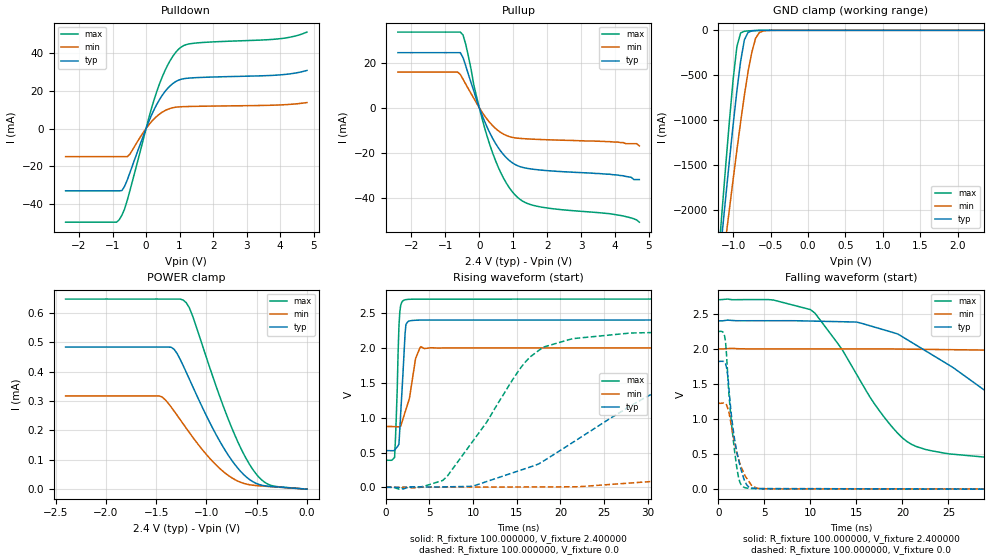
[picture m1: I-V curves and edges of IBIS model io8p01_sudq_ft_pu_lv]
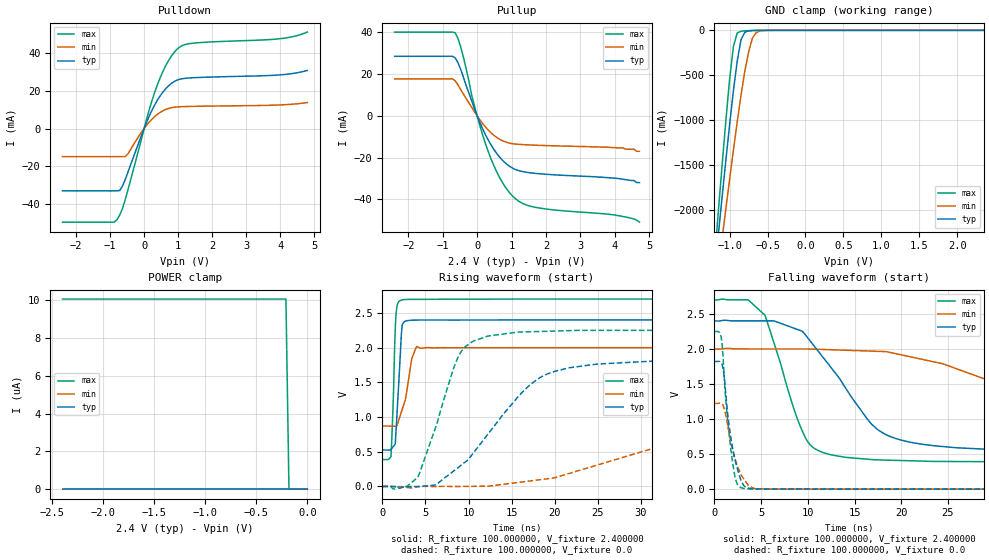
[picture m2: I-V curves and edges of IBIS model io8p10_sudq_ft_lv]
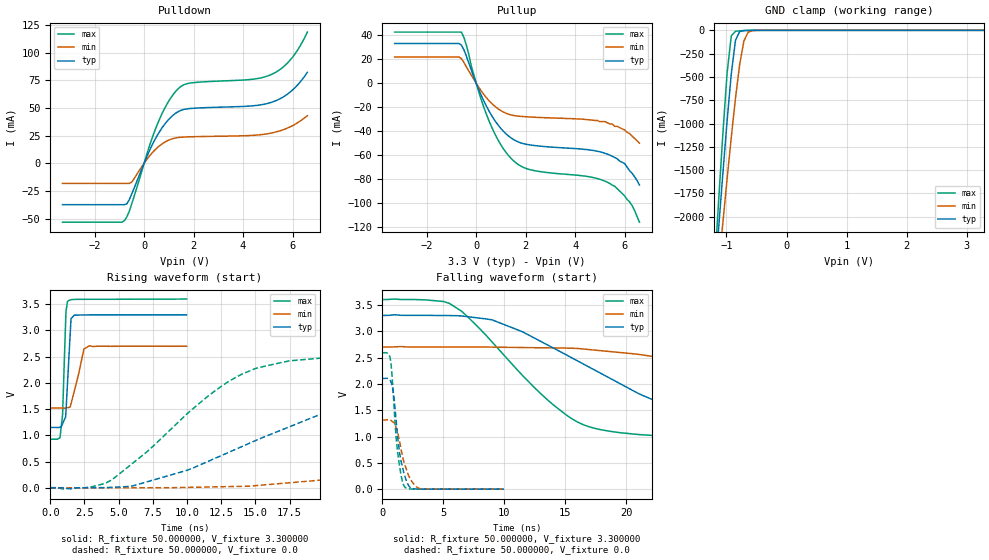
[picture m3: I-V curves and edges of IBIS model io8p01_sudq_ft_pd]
| IBIS file stm32f303x6x8_334_wlcsp49.ibs
[IBIS ver] 4.2
[File name] stm32f303x6x8_334_wlcsp49.ibs
[File Rev] 1
[Date]  29-09-2025
[Source] Data Created at STMicroelectronics
[Notes]  File originated from ELDO simulations.
[Disclaimer]  This information is for modeling purpose only and is
   not guaranted. The information is subject to change without
   notice.
[Copyright] Copyright 2025 STMicroelectronics Inc.
|   Component stm32f303x6x8_334_wlcsp49
[Component] stm32f303x6x8_334_wlcsp49
[Manufacturer] STMicroelectronics
[Package]
| variable   typ   min   max
R_pkg   0.0   0.0   0.0
L_pkg   0.0H   0.0H   0.0H
C_pkg   0.0F   0.0F   0.0F
[Pin]  signal_name   model_name   R_pin   L_pin   C_pin
A1 PA14 io8p_wsudqh_i2c_ft
A2 PA15 io8p_wsudqh_i2c_ft
A3 PB3 io8p_sudq_ft
A4 PB6 io8p_wsudqh_i2c_ft
A5 BOOT0 vpp_test_hv
A6 PB9 io8p_wsudqh_i2c_ft
A7 VDD POWER
B1 VSS GND
B2 VDD POWER
B3 PB4 io8p_sudq_ft
B4 PB5 io8p_sudq_ft
B5 PB7 io8p_wsudqh_i2c_ft
B6 PB8 io8p_wsudqh_i2c_ft
B7 VSS GND
C1 PA11 io8p_sudq_ft
C2 PA13 io8p_sudq_ft
C3 PA12 io8p_sudq_ft
C4 PA10 io8p_sudq_ft
C5 PC3 io8p_sudq_tc
C6 PF1 io8p_sudq_ft
C7 PF0 io8p_sudq_ft
D1 PA8 io8p_sudq_ft
D2 PA9 io8p_sudq_ft
D3 PB15 io8p_sudq_tc
D4 PC7 io8p_sudq_ft
D5 PA2 io8p_sudq_tc
D6 PA0 io8p_sudq_tc
D7 NRST ioreset_tc_v33
E1 PB14 io8p_sudq_tc
E2 PB13 io8p_sudq_tc
E3 PC5 io8p_sudq_tc
E4 PA6 io8p_sudq_tc
E5 PA3 io8p_sudq_tc
E6 VDDA POWER
E7 VSSA GND
F1 PB12 io8p_sudq_tc
F2 PB2 io8p_sudq_tc
F3 PB0 io8p_sudq_tc
F4 PA7 io8p_sudq_tc
F5 PA4 io8p_sudq_tc
F6 VSS GND
F7 VREFP POWER
G1 PB11 io8p_sudq_tc
G2 PB10 io8p_sudq_tc
G3 PB1 io8p_sudq_tc
G4 PC4 io8p_sudq_tc
G5 PA5 io8p_sudq_tc
G6 VDD POWER
G7 PA1 io8p_sudq_tc
[Model Selector] io8p_sudq_ft
io8p01_sudq_ft_pd_lv  "SPEED01 2P0V, PD=40kOhm"
io8p01_sudq_ft_pu_lv  "SPEED01 2P0V, PU=40kOhm"
io8p01_sudq_ft_lv  "SPEED01 2P0V"
io8p10_sudq_ft_pd_lv  "SPEED10 2P0V, PD=40kOhm"
io8p10_sudq_ft_pu_lv  "SPEED10 2P0V, PU=40kOhm"
io8p10_sudq_ft_lv  "SPEED10 2P0V"
io8p11_sudq_ft_pd_lv  "SPEED11 2P0V, PD=40kOhm"
io8p11_sudq_ft_pu_lv  "SPEED11 2P0V, PU=40kOhm"
io8p11_sudq_ft_lv  "SPEED11 2P0V"
io8p01_sudq_ft_pd  "SPEED01, PD=40kOhm"
io8p01_sudq_ft_pu  "SPEED01, PU=40kOhm"
io8p01_sudq_ft  "SPEED01"
io8p10_sudq_ft_pd  "SPEED10, PD=40kOhm"
io8p10_sudq_ft_pu  "SPEED10, PU=40kOhm"
io8p10_sudq_ft  "SPEED10"
io8p11_sudq_ft_pd  "SPEED11, PD=40kOhm"
io8p11_sudq_ft_pu  "SPEED11, PU=40kOhm"
io8p11_sudq_ft  "SPEED11"
[Model Selector] io8p_sudq_tc
io8p01_sudq_tc_pd_lv  "SPEED01 2P0V, PD=40kOhm"
io8p01_sudq_tc_pu_lv  "SPEED01 2P0V, PU=40kOhm"
io8p01_sudq_tc_lv  "SPEED01 2P0V"
io8p10_sudq_tc_pd_lv  "SPEED10 2P0V, PD=40kOhm"
io8p10_sudq_tc_pu_lv  "SPEED10 2P0V, PU=40kOhm"
io8p10_sudq_tc_lv  "SPEED10 2P0V"
io8p11_sudq_tc_pd_lv  "SPEED11 2P0V, PD=40kOhm"
io8p11_sudq_tc_pu_lv  "SPEED11 2P0V, PU=40kOhm"
io8p11_sudq_tc_lv  "SPEED11 2P0V"
io8p01_sudq_tc_pd  "SPEED01, PD=40kOhm"
io8p01_sudq_tc_pu  "SPEED01, PU=40kOhm"
io8p01_sudq_tc  "SPEED01"
io8p10_sudq_tc_pd  "SPEED10, PD=40kOhm"
io8p10_sudq_tc_pu  "SPEED10, PU=40kOhm"
io8p10_sudq_tc  "SPEED10"
io8p11_sudq_tc_pd  "SPEED11, PD=40kOhm"
io8p11_sudq_tc_pu  "SPEED11, PU=40kOhm"
io8p11_sudq_tc  "SPEED11"
[Model Selector] io8p_wsudqh_i2c_ft
io8p_wsudqh_i2c_ft_lv_pd  "General purpose IO with I2C capability on. 5V tolerant. 1.8V range with pull down"
io8p_wsudqh_i2c_ft_lv_pu  "General purpose IO with I2C capability on. 5V tolerant. 1.8V range with pull up"
io8p_wsudqh_i2c_ft_lv  "General purpose IO with I2C capability on. 5V tolerant. 1.8V range"
io8p_wsudqh_i2c_ft_pd  "General purpose IO with I2C capability on. 5V tolerant. 3.3V range with pull down"
io8p_wsudqh_i2c_ft_pu  "General purpose IO with I2C capability on. 5V tolerant. 3.3V range with pull up"
io8p_wsudqh_i2c_ft_i2c  "General purpose IO with I2C capability on. 5V tolerant. 3.3V range"
[Model Selector] ioreset_tc_v33
ioreset_tc_v33_pu_lv  "IORESET 2V + PU=40kOhm"
ioreset_tc_v33_nopu_lv  "IORESET 2V"
ioreset_tc_v33_pu  "IORESET + PU=40kOhm"
ioreset_tc_v33_nopu  "IORESET"
[Model Selector] vpp_test_hv
vpp_test_hv_3p3  "Input Buffer"
vpp_test_hv_2p4  "Input Buffer 2P0V"
| Models and submodels in the file (48): io8p01_sudq_ft_pd_lv (I/O), io8p01_sudq_ft_pu_lv (I/O), io8p01_sudq_ft_lv (I/O), io8p10_sudq_ft_pd_lv (I/O), io8p10_sudq_ft_pu_lv (I/O), io8p10_sudq_ft_lv (I/O), io8p11_sudq_ft_pd_lv (I/O), io8p11_sudq_ft_pu_lv (I/O), io8p11_sudq_ft_lv (I/O), io8p01_sudq_ft_pd (I/O), io8p01_sudq_ft_pu (I/O), io8p01_sudq_ft (I/O), io8p10_sudq_ft_pd (I/O), io8p10_sudq_ft_pu (I/O), io8p10_sudq_ft (I/O), io8p11_sudq_ft_pd (I/O), io8p11_sudq_ft_pu (I/O), io8p11_sudq_ft (I/O), io8p01_sudq_tc_pd_lv (I/O), io8p01_sudq_tc_pu_lv (I/O), io8p01_sudq_tc_lv (I/O), io8p10_sudq_tc_pd_lv (I/O), io8p10_sudq_tc_pu_lv (I/O), io8p10_sudq_tc_lv (I/O), io8p11_sudq_tc_pd_lv (I/O), io8p11_sudq_tc_pu_lv (I/O), io8p11_sudq_tc_lv (I/O), io8p01_sudq_tc_pd (I/O), io8p01_sudq_tc_pu (I/O), io8p01_sudq_tc (I/O), io8p10_sudq_tc_pd (I/O), io8p10_sudq_tc_pu (I/O), io8p10_sudq_tc (I/O), io8p11_sudq_tc_pd (I/O), io8p11_sudq_tc_pu (I/O), io8p11_sudq_tc (I/O), io8p_wsudqh_i2c_ft_lv_pd (I/O), io8p_wsudqh_i2c_ft_lv_pu (I/O), io8p_wsudqh_i2c_ft_lv (I/O), io8p_wsudqh_i2c_ft_pd (I/O), io8p_wsudqh_i2c_ft_pu (I/O), io8p_wsudqh_i2c_ft_i2c (I/O), ioreset_tc_v33_pu_lv (I/O_open_drain), ioreset_tc_v33_nopu_lv (I/O_open_drain), ioreset_tc_v33_pu (I/O_open_drain), ioreset_tc_v33_nopu (I/O_open_drain), vpp_test_hv_2p4 (Input), vpp_test_hv_3p3 (Input)
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|   Model io8p01_sudq_ft_pu_lv
[Model]  io8p01_sudq_ft_pu_lv
Model_type I/O
Polarity   Non-Inverting
Enable   Active-Low
Vinl =   0.720000V
Vinh =   1.680000V
Vmeas =  1.200000V
Cref =   50.000000pF
Rref =   100.000000M
Vref =   0.0V
C_comp   1.970100pF   1.887900pF   2.069400pF
[Temperature Range]   25.000000   0.125000k   -40.000000
[Pullup Reference]   2.400000V   2.000000V   2.700000V
[Pulldown Reference]   0.0V   0.0V   0.0V
[POWER Clamp Reference]   2.400000V   2.000000V   2.700000V
[GND Clamp Reference]   0.0V   0.0V   0.0V
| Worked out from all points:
|   slope of the pulldown table from 0 to 0.36 V, typ, clamps not added: 25.5 ohm
|   slope of the pullup table from 0 to 0.36 V, typ, clamps not added: 28.4 ohm
|   GND clamp passes 1 mA (typ) near -0.64 V on its own axis
|   rising waveform, R_fixture 100.000000, V_fixture 2.400000: 20-80 % time 497ps typ, 1.06ns min, 335ps max; typ from 0.527 V to 2.4 V
|   rising waveform, R_fixture 100.000000, V_fixture 0.0: 20-80 % time 14.6ns typ, 42.8ns min, 7.27ns max; typ from 0.001 V to 1.82 V
|   falling waveform, R_fixture 100.000000, V_fixture 2.400000: 20-80 % time 12.9ns typ, 32.5ns min, 7.06ns max; typ from 2.4 V to 0.527 V
|   falling waveform, R_fixture 100.000000, V_fixture 0.0: 20-80 % time 1.16ns typ, 1.4ns min, 913ps max; typ from 1.82 V to 0.001 V
[Pulldown]
|Voltage   I(typ)   I(min)   I(max)
-2.4V     -33.16mA   -14.98mA   -49.86mA
-880mV    -33.16mA   -14.98mA   -49.86mA
-800mV    -33.16mA   -14.98mA   -48.55mA
-640mV    -30.75mA   -14.98mA   -42.77mA
-480mV    -23.43mA   -13.57mA   -32.92mA
80mV      3.651mA    1.905mA    5.506mA
400mV     15.37mA    7.665mA    23.73mA
720mV     22.75mA    10.69mA    36.23mA
1.04V     26.18mA    11.57mA    43.27mA
1.52V     27.09mA    11.81mA    45.55mA
4V        28.55mA    12.55mA    47.81mA
4.8V      30.9mA     13.81mA    51.31mA
[Pullup]
|Voltage   I(typ)   I(min)   I(max)
-2.4V     24.57mA    15.91mA    33.73mA
-640mV    24.57mA    15.91mA    33.73mA
-480mV    22.32mA    12.71mA    32.43mA
-400mV    18.71mA    10.52mA    28.28mA
-160mV    7.421mA    4.162mA    10.02mA
0V        81fA       15.2pA     0A
320mV     -11.51mA   -6.781mA   -16.98mA
720mV     -21mA      -11.8mA    -31.53mA
1.2V      -26.24mA   -13.65mA   -40.83mA
1.76V     -27.69mA   -14.12mA   -44.07mA
3.84V     -29.6mA    -15.1mA    -47.2mA
4.72V     -32mA      -17mA      -51mA
[GND_clamp]
|Voltage   I(typ)   I(min)   I(max)
-2.4V     -9.788A    -9.782A    -9.734A
-1.2V     -2.718A    -3.02A     -2.568A
-1.15V    -2.29A     -2.675A    -2.036A
-1.1V     -1.868A    -2.333A    -1.515A
-1.05V    -1.454A    -1.995A    -1.012A
-950mV    -674.5mA   -1.337A    -180.5mA
-900mV    -345.2mA   -1.023A    -29.72mA
-850mV    -106.4mA   -726mA     -10.13mA
-750mV    -6.396mA   -244mA     -4.026mA
-700mV    -2.558mA   -88.61mA   -2.329mA
-600mV    -416uA     -7.739mA   -368uA
2.35V     0A         0A         0A
[POWER_clamp]
|Voltage   I(typ)   I(min)   I(max)
-2.4V     483.8uA    317.4uA    647uA
-1.47V    483.8uA    317.4uA    647uA
-1.32V    475.6uA    265.2uA    647uA
-1.23V    419.7uA    221.6uA    643.3uA
-1.17V    374.8uA    192.7uA    617.6uA
-1.14V    352.1uA    178.7uA    591.9uA
-840mV    147uA      62.15uA    289.6uA
-690mV    72.24uA    27.76uA    162.7uA
-540mV    25.74uA    13.55uA    67.63uA
-450mV    13.38uA    10.75uA    31.36uA
-360mV    9.231uA    8.535uA    12.97uA
0V        0A         0A         0A
[Ramp]
| variable   typ   min   max
dV/dt_r  1.09269/14.55881n   0.73353/42.71845n   1.34908/7.26325n
dV/dt_f  1.12400/12.83842n   0.67649/32.44923n   1.38689/7.04961n
R_load = 100.000000
[Rising Waveform]
R_fixture= 100.000000
V_fixture= 2.400000
V_fixture_min= 2.000000
V_fixture_max= 2.700000
|time   V(typ)   V(min)   V(max)
0s        526.5mV    872.5mV    388.6mV
1.001ns   534.8mV    870.7mV    429.3mV
1.301ns   581.8mV    869.1mV    1.401V
1.502ns   620.7mV    868.5mV    2.316V
1.602ns   841mV      868.2mV    2.522V
2.102ns   1.968V     1.038V     2.685V
2.302ns   2.337V     1.118V     2.692V
3.403ns   2.396V     1.846V     2.698V
4.004ns   2.398V     2.018V     2.698V
49.85ns   2.4V       2V         2.7V
[Rising Waveform]
R_fixture= 100.000000
V_fixture= 0.0
V_fixture_min= 0.0
V_fixture_max= 0.0
|time   V(typ)   V(min)   V(max)
0s        1.057mV    1.357mV    941.6uV
6.507ns   6.739mV    4.851mV    98.8mV
15.52ns   249.4mV    5.766mV    1.725V
18.02ns   374.6mV    6.657mV    2.009V
28.03ns   1.166V     62.6mV     2.213V
34.53ns   1.553V     120.9mV    2.23V
43.04ns   1.725V     229mV      2.248V
79.08ns   1.822V     883.8mV    2.25V
103.1ns   1.822V     1.116V     2.249V
249.2ns   1.822V     1.224V     2.25V
[Falling Waveform]
R_fixture= 100.000000
V_fixture= 2.400000
V_fixture_min= 2.000000
V_fixture_max= 2.700000
|time   V(typ)   V(min)   V(max)
0s        2.4V       2V         2.7V
10.01ns   2.397V     2V         2.56V
15.02ns   2.383V     2V         1.64V
20.02ns   2.171V     1.997V     729.2mV
29.53ns   1.353V     1.982V     451.1mV
38.04ns   762.8mV    1.926V     413.2mV
57.06ns   576.4mV    1.555V     391.8mV
84.58ns   537.8mV    1.049V     388.5mV
102.6ns   530.3mV    958.5mV    388.5mV
249.2ns   526.5mV    872.5mV    388.6mV
[Falling Waveform]
R_fixture= 100.000000
V_fixture= 0.0
V_fixture_min= 0.0
V_fixture_max= 0.0
|time   V(typ)   V(min)   V(max)
0s        1.822V     1.224V     2.25V
700.7ps   1.803V     1.224V     2.18V
800.8ps   1.785V     1.217V     2.098V
1.001ns   1.655V     1.167V     1.705V
1.401ns   1.091V     924.7mV    994.1mV
1.802ns   692.7mV    650.1mV    517.8mV
2.302ns   370.4mV    389.6mV    121.1mV
2.903ns   110.3mV    193.7mV    21.86mV
4.605ns   7.762mV    8.133mV    8.175mV
49.85ns   1.057mV    1.357mV    941.6uV
|   Model io8p10_sudq_ft_lv
[Model]  io8p10_sudq_ft_lv
Model_type I/O
Polarity   Non-Inverting
Enable   Active-Low
Vinl =   0.720000V
Vinh =   1.680000V
Vmeas =  1.200000V
Cref =   50.000000pF
Rref =   100.000000M
Vref =   0.0V
C_comp   1.970100pF   1.887900pF   2.069400pF
[Temperature Range]   25.000000   0.125000k   -40.000000
[Pullup Reference]   2.400000V   2.000000V   2.700000V
[Pulldown Reference]   0.0V   0.0V   0.0V
[POWER Clamp Reference]   2.400000V   2.000000V   2.700000V
[GND Clamp Reference]   0.0V   0.0V   0.0V
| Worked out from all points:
|   slope of the pulldown table from 0 to 0.36 V, typ, clamps not added: 25.5 ohm
|   slope of the pullup table from 0 to 0.36 V, typ, clamps not added: 28.4 ohm
|   GND clamp passes 1 mA (typ) near -0.64 V on its own axis
|   rising waveform, R_fixture 100.000000, V_fixture 2.400000: 20-80 % time 501ps typ, 1.06ns min, 336ps max; typ from 0.525 V to 2.4 V
|   rising waveform, R_fixture 100.000000, V_fixture 0.0: 20-80 % time 7.32ns typ, 21.7ns min, 3.52ns max; typ from 0 V to 1.82 V
|   falling waveform, R_fixture 100.000000, V_fixture 2.400000: 20-80 % time 6.27ns typ, 18.5ns min, 3.33ns max; typ from 2.4 V to 0.525 V
|   falling waveform, R_fixture 100.000000, V_fixture 0.0: 20-80 % time 1.16ns typ, 1.4ns min, 914ps max; typ from 1.82 V to 0 V
[Pulldown]
|Voltage   I(typ)   I(min)   I(max)
-2.4V     -33.16mA   -14.98mA   -49.86mA
-880mV    -33.16mA   -14.98mA   -49.86mA
-800mV    -33.16mA   -14.98mA   -48.55mA
-640mV    -30.75mA   -14.98mA   -42.76mA
-480mV    -23.43mA   -13.57mA   -32.92mA
80mV      3.651mA    1.905mA    5.506mA
400mV     15.37mA    7.665mA    23.73mA
720mV     22.75mA    10.69mA    36.23mA
1.04V     26.18mA    11.57mA    43.27mA
1.52V     27.09mA    11.81mA    45.55mA
4V        28.55mA    12.55mA    47.81mA
4.8V      30.9mA     13.81mA    51.31mA
[Pullup]
|Voltage   I(typ)   I(min)   I(max)
-2.4V     28.57mA    17.75mA    40.17mA
-720mV    28.57mA    17.75mA    40.17mA
-640mV    27.85mA    16.83mA    39.88mA
-480mV    22.38mA    12.65mA    33.22mA
-80mV     3.427mA    2.066mA    4.957mA
160mV     -6.219mA   -3.715mA   -9.137mA
320mV     -11.51mA   -6.781mA   -16.98mA
720mV     -21mA      -11.8mA    -31.54mA
1.12V     -25.77mA   -13.54mA   -39.82mA
1.76V     -27.69mA   -14.12mA   -44.07mA
4V        -29.9mA    -15.2mA    -47.5mA
4.72V     -32mA      -17mA      -51mA
[GND_clamp]
|Voltage   I(typ)   I(min)   I(max)
-2.4V     -9.788A    -9.782A    -9.734A
-1.2V     -2.718A    -3.02A     -2.568A
-1.15V    -2.29A     -2.675A    -2.036A
-1.1V     -1.868A    -2.333A    -1.515A
-1.05V    -1.454A    -1.995A    -1.012A
-950mV    -674.5mA   -1.337A    -180.5mA
-900mV    -345.2mA   -1.023A    -29.72mA
-850mV    -106.4mA   -726mA     -10.13mA
-750mV    -6.396mA   -244mA     -4.026mA
-700mV    -2.558mA   -88.61mA   -2.329mA
-600mV    -416uA     -7.739mA   -368uA
2.35V     0A         0A         0A
[POWER_clamp]
|Voltage   I(typ)   I(min)   I(max)
-2.4V     0A         0A         10.06uA
-210mV    0A         0A         10.06uA
-180mV    0A         0A         0A
0V        0A         0A         0A
[Ramp]
| variable   typ   min   max
dV/dt_r  1.09308/7.31082n   0.73308/21.71145n   1.34964/3.51759n
dV/dt_f  1.12481/6.26349n   0.67631/18.49686n   1.38754/3.32485n
R_load = 100.000000
[Rising Waveform]
R_fixture= 100.000000
V_fixture= 2.400000
V_fixture_min= 2.000000
V_fixture_max= 2.700000
|time   V(typ)   V(min)   V(max)
0s        525.2mV    870.3mV    387.4mV
1.001ns   533.2mV    868.7mV    426.9mV
1.301ns   579.1mV    867.1mV    1.388V
1.502ns   617.1mV    866.5mV    2.304V
1.702ns   1.054V     877mV      2.604V
2.202ns   2.189V     1.072V     2.684V
2.603ns   2.379V     1.227V     2.693V
3.403ns   2.395V     1.838V     2.696V
4.004ns   2.397V     2.017V     2.696V
49.85ns   2.4V       2V         2.7V
[Rising Waveform]
R_fixture= 100.000000
V_fixture= 0.0
V_fixture_min= 0.0
V_fixture_max= 0.0
|time   V(typ)   V(min)   V(max)
0s        1.81nV     16.19nV    1.388nV
2.803ns   -3.281mV   -14.07mV   -1.578mV
4.204ns   -1.834mV   -2.504mV   153.3mV
8.809ns   274.6mV    -1.375mV   1.87V
12.21ns   748.9mV    4.656mV    2.166V
18.02ns   1.547V     92.84mV    2.232V
24.82ns   1.763V     304.5mV    2.249V
40.24ns   1.817V     861.6mV    2.249V
51.85ns   1.822V     1.107V     2.249V
99.7ns    1.822V     1.223V     2.249V
[Falling Waveform]
R_fixture= 100.000000
V_fixture= 2.400000
V_fixture_min= 2.000000
V_fixture_max= 2.700000
|time   V(typ)   V(min)   V(max)
0s        2.4V       2V         2.7V
3.604ns   2.401V     2V         2.703V
5.405ns   2.402V     2V         2.482V
9.81ns    2.189V     2V         715.2mV
14.01ns   1.448V     1.982V     453.6mV
18.22ns   786.7mV    1.963V     414.6mV
25.83ns   591.3mV    1.722V     393.9mV
36.04ns   545.2mV    1.277V     387.5mV
53.05ns   528.1mV    942.3mV    387.4mV
99.7ns    525.2mV    870.3mV    387.4mV
[Falling Waveform]
R_fixture= 100.000000
V_fixture= 0.0
V_fixture_min= 0.0
V_fixture_max= 0.0
|time   V(typ)   V(min)   V(max)
0s        1.822V     1.223V     2.249V
700.7ps   1.802V     1.222V     2.18V
800.8ps   1.785V     1.215V     2.098V
1.001ns   1.656V     1.165V     1.707V
1.401ns   1.093V     924.2mV    997.1mV
1.902ns   616.8mV    592mV      421.8mV
2.302ns   368.5mV    388.7mV    122.4mV
2.903ns   107.4mV    191.2mV    17.72mV
4.705ns   2.748mV    4.47mV     1.93mV
49.85ns   1.81nV     16.19nV    1.388nV
|   Model io8p01_sudq_ft_pd
[Model]  io8p01_sudq_ft_pd
Model_type I/O
Polarity   Non-Inverting
Enable   Active-Low
Vinl =   0.990000V
Vinh =   2.310000V
Vmeas =  1.650000V
Cref =   50.000000pF
Rref =   100.000000M
Vref =   0.0V
C_comp   1.970900pF   1.892300pF   2.063200pF
[Temperature Range]   25.000000   0.125000k   -40.000000
[Pullup Reference]   3.300000V   2.700000V   3.600000V
[Pulldown Reference]   0.0V   0.0V   0.0V
[POWER Clamp Reference]   3.300000V   2.700000V   3.600000V
[GND Clamp Reference]   0.0V   0.0V   0.0V
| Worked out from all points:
|   slope of the pulldown table from 0 to 0.495 V, typ, clamps not added: 20.9 ohm
|   slope of the pullup table from 0 to 0.495 V, typ, clamps not added: 22.2 ohm
|   GND clamp passes 1 mA (typ) near -0.64 V on its own axis
|   rising waveform, R_fixture 50.000000, V_fixture 3.300000: 20-80 % time 269ps typ, 640ps min, 200ps max; typ from 1.15 V to 3.3 V
|   rising waveform, R_fixture 50.000000, V_fixture 0.0: 20-80 % time 12.6ns typ, 30.4ns min, 7.07ns max; typ from 0 V to 2.1 V
|   falling waveform, R_fixture 50.000000, V_fixture 3.300000: 20-80 % time 11ns typ, 22.7ns min, 6.9ns max; typ from 3.3 V to 1.15 V
|   falling waveform, R_fixture 50.000000, V_fixture 0.0: 20-80 % time 664ps typ, 860ps min, 541ps max; typ from 2.1 V to 0 V
[Pulldown]
|Voltage   I(typ)   I(min)   I(max)
-3.3V     -37.45mA   -18.2mA    -53.24mA
-800mV    -37.45mA   -18.2mA    -51.9mA
-700mV    -36.7mA    -18.2mA    -48.48mA
-500mV    -27.71mA   -17.01mA   -36.66mA
200mV     10.57mA    6.084mA    14.57mA
500mV     23.91mA    13.38mA    33.24mA
900mV     37.17mA    19.88mA    52.48mA
1.3V      45.55mA    23.01mA    65.5mA
1.8V      49.29mA    23.83mA    72.18mA
5.1V      54.68mA    27.07mA    79.72mA
5.9V      64.2mA     32.82mA    93.01mA
6.6V      82.13mA    42.97mA    118.5mA
[Pullup]
|Voltage   I(typ)   I(min)   I(max)
-3.3V     33.17mA    21.9mA     42.7mA
-600mV    31.87mA    20.58mA    42.7mA
-400mV    22.79mA    13.76mA    31.9mA
100mV     -5.13mA    -3.299mA   -6.952mA
500mV     -22.5mA    -14.16mA   -30.52mA
900mV     -35.28mA   -21.55mA   -48mA
1.4V      -45.55mA   -26.41mA   -62.54mA
2.2V      -51.57mA   -28.22mA   -72.25mA
5.3V      -59.1mA    -33mA      -82.6mA
6V        -67mA      -39mA      -94mA
6.2V      -73mA      -42mA      -99mA
6.6V      -85mA      -50mA      -116mA
[GND_clamp]
|Voltage   I(typ)   I(min)   I(max)
-3.3V     -9.525A    -9.501A    -9.513A
-1.2V     -2.719A    -3.023A    -2.568A
-1.13V    -2.122A    -2.541A    -1.826A
-1.06V    -1.537A    -2.065A    -1.111A
-990mV    -975.7mA   -1.599A    -462mA
-920mV    -467.5mA   -1.149A    -59.02mA
-850mV    -106.6mA   -727.3mA   -10.13mA
-780mV    -13.08mA   -365.4mA   -5.271mA
-710mV    -3.06mA    -114.8mA   -2.651mA
-640mV    -957.2uA   -20.17mA   -921.6uA
-570mV    -212.9uA   -3.969mA   -172uA
3.28V     83.81uA    63.75uA    93.54uA
[POWER_clamp]
|Voltage   I(typ)   I(min)   I(max)
-3.28V    0A         0A         0A
0V        0A         0A         0A
[Ramp]
| variable   typ   min   max
dV/dt_r  1.26156/12.54362n   0.78870/30.38144n   1.55370/7.05539n
dV/dt_f  1.28928/10.94568n   0.70680/22.67171n   1.60430/6.89156n
R_load = 50.000000
[Rising Waveform]
R_fixture= 50.000000
V_fixture= 3.300000
V_fixture_min= 2.700000
V_fixture_max= 3.600000
|time   V(typ)   V(min)   V(max)
0s        1.15V      1.52V      925.1mV
720.7ps   1.152V     1.52V      978.8mV
900.9ps   1.221V     1.519V     1.392V
1.141ns   1.421V     1.522V     3.31V
1.261ns   1.999V     1.527V     3.552V
1.522ns   3.227V     1.604V     3.586V
1.762ns   3.293V     1.85V      3.592V
2.462ns   3.296V     2.645V     3.594V
2.863ns   3.297V     2.708V     3.595V
9.97ns    3.299V     2.699V     3.599V
[Rising Waveform]
R_fixture= 50.000000
V_fixture= 0.0
V_fixture_min= 0.0
V_fixture_max= 0.0
|time   V(typ)   V(min)   V(max)
0s        1.98nV     11.35nV    2.495nV
4.505ns   8.245mV    25.84uV    149.8mV
10.01ns   333.1mV    6.62mV     1.412V
14.01ns   784.8mV    26.04mV    2.166V
17.52ns   1.165V     95.18mV    2.421V
22.02ns   1.586V     194.8mV    2.524V
32.03ns   1.987V     468.3mV    2.582V
55.56ns   2.099V     1.053V     2.59V
75.08ns   2.102V     1.238V     2.59V
249.2ns   2.102V     1.315V     2.59V
[Falling Waveform]
R_fixture= 50.000000
V_fixture= 3.300000
V_fixture_min= 2.700000
V_fixture_max= 3.600000
|time   V(typ)   V(min)   V(max)
0s        3.299V     2.699V     3.599V
5.506ns   3.296V     2.699V     3.527V
9.009ns   3.215V     2.697V     2.794V
13.51ns   2.743V     2.683V     1.704V
16.52ns   2.374V     2.661V     1.221V
24.52ns   1.517V     2.439V     989.5mV
32.53ns   1.278V     2.152V     947.7mV
42.04ns   1.2V       1.835V     933.5mV
70.57ns   1.156V     1.581V     925mV
249.2ns   1.15V      1.52V      925.1mV
[Falling Waveform]
R_fixture= 50.000000
V_fixture= 0.0
V_fixture_min= 0.0
V_fixture_max= 0.0
|time   V(typ)   V(min)   V(max)
0s        2.102V     1.315V     2.59V
660.7ps   2.06V      1.314V     2.464V
900.9ps   1.839V     1.271V     1.793V
1.141ns   1.272V     1.163V     949.5mV
1.261ns   974.3mV    1.073V     691.1mV
1.602ns   461.9mV    684.2mV    189.4mV
1.862ns   235.9mV    450.5mV    34.15mV
2.282ns   33.01mV    202.5mV    4.353mV
3.103ns   1.374mV    10.53mV    452.6uV
9.97ns    1.98nV     11.35nV    2.495nV
